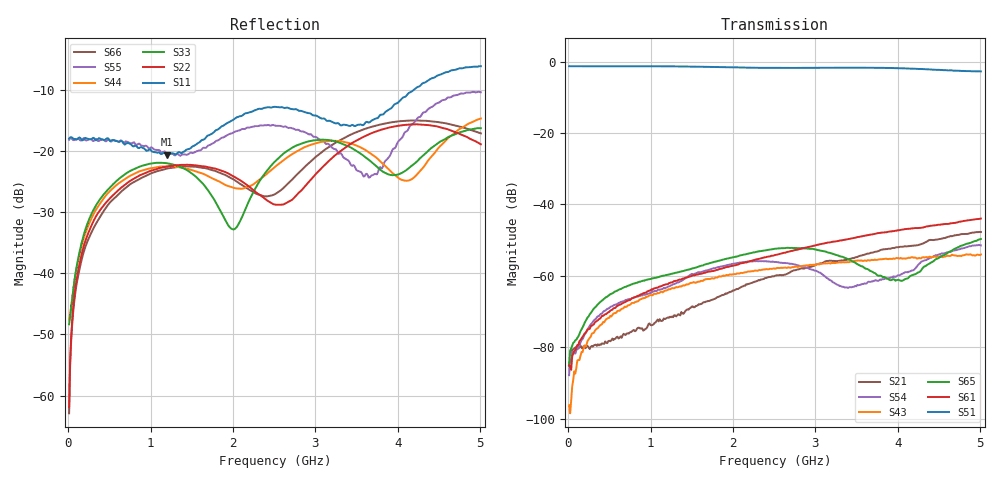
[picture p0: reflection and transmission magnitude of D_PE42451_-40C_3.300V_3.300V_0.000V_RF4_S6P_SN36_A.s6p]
! Device ID: PE42451
! Serial: 36
! Insertion: A
! Temp: -40C
! VDD: 3.300
! Control_Hi: 100.000
! Control_Lo: 0.000
! Logic State: RF4
! Port 1: RFC
! Port 2: RF1
! Port 3: RF2
! Port 4: RF3
! Port 5: RF4
! Port 6: RF5
! V1 = 0.00
! V2 = 0.00
! V3 = 3.30
! V4 = 0.00
! IDD: 1.607110e-05
#  Hz  S  RI  R  50
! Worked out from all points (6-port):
!   401 points, 10 MHz to 5.01 GHz, reference 50 ohm
!   strongest paths, dB at 10 MHz, 1.26 GHz, 2.51 GHz, 3.76 GHz, 5.01 GHz:
!     S51: -1.3, -1.3, -1.8, -1.7, -2.7
!     S61: -85.1, -61.9, -54.2, -48.0, -44.0
!     S65: -85.2, -59.4, -52.4, -59.9, -49.7
!     S43: -96.2, -63.4, -58.0, -55.4, -54.0
!     S54: -87.8, -62.6, -56.1, -61.4, -51.4
!     S21: -84.3, -71.4, -60.0, -53.1, -47.7
!   lowest |S11| = -20.7 dB at 1.198 GHz (marker M1), VSWR 1.20, Z = 55 - j8.39 ohm
!   |S11| at or under -10 dB: start of sweep to 4.198 GHz
